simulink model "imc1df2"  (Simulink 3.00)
settings: Solver=ode45  SolverMode=SingleTasking  StartTime=0.0  StopTime=50  MaxStep=st_size  RelTol=1e-5  AbsTol=1e-6
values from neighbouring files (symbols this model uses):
  d_through_p = get(MAIN_MENU(19),'Value')    [cback.m]    (also in imcmenu.m = 0)
  Disturb = Setpoint    [mimo_MSF1DF_sim.m]    (also in mimo_MSF2DF_sim.m)
  Satlb = temp1    [cback.m]    (also in imcmenu.m = str2num(satlbs))
  Satub = temp1    [cback.m]    (also in imcmenu.m = str2num(satubs))
  Setpoint = zeros(1,n)    [mimo_MSF1DF_sim.m]    (also in mimo_MSF2DF_sim.m)
undefined symbols (not defined in the file or in its folder): denCs, denPd, mdeadx, numCs, numPd, pdeadx, XdenMs, XdenPs, XnumMs, XnumPs

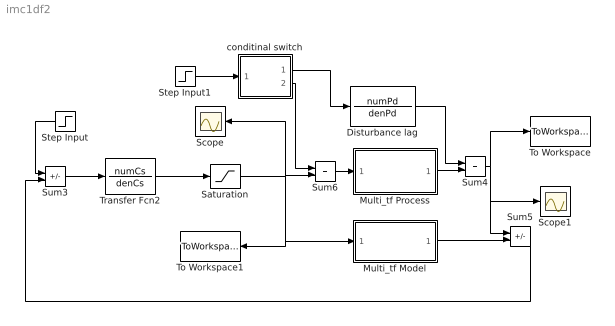
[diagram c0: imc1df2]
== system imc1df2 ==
  Disturbance lag : TransferFcn  Numerator=numPd  Denominator=denPd
  Multi_tf Model : Subsystem
  Multi_tf Process : Subsystem
  Saturation : Saturate  UpperLimit=Satub  LowerLimit=Satlb
  Scope : Scope
  Scope1 : Scope
  Step Input : Step  Orientation=left  Time=0  Before=0  After=Setpoint  SampleTime=0
  Step Input1 : Step  Time=0  Before=0  After=Disturb  SampleTime=0
  Sum3 : Sum  Inputs=+-  SaturateOnIntegerOverflow=on
  Sum4 : Sum  Inputs=++  SaturateOnIntegerOverflow=on
  Sum5 : Sum  Inputs=+-  SaturateOnIntegerOverflow=on
  Sum6 : Sum  Inputs=++  SaturateOnIntegerOverflow=on
  To Workspace : ToWorkspace  VariableName=simout  SampleTime=-1  SaveFormat=Matrix
  To Workspace1 : ToWorkspace  VariableName=effort  SampleTime=-1  SaveFormat=Matrix
  Transfer Fcn2 : TransferFcn  Numerator=numCs  Denominator=denCs
  conditinal switch : Subsystem  Description=pass input signal through out1 if condition is true.
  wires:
  Sum3/1 -> Transfer Fcn2/1
  Transfer Fcn2/1 -> Saturation/1
  Step Input/1 -> Sum3/1
  Sum5/1 -> Sum3/2
  Multi_tf Model/1(Out1) -> Sum5/2
  Disturbance lag/1 -> Sum4/1
  Step Input1/1 -> conditinal switch/1(In)
  conditinal switch/1(Out2) -> Disturbance lag/1
  Saturation/1 -> Sum6/2, Multi_tf Model/1(In1), Scope/1, To Workspace1/1
  conditinal switch/2(Out1) -> Sum6/1
  Sum6/1 -> Multi_tf Process/1(In1)
  Multi_tf Process/1(Out1) -> Sum4/2
  Sum4/1 -> Sum5/1, To Workspace/1, Scope1/1

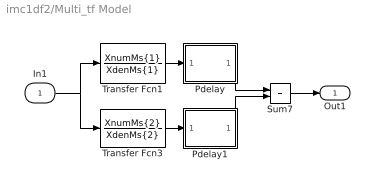
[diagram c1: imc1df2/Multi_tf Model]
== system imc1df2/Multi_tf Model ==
  In1 : Inport  Port=1  PortWidth=-1  SampleTime=-1  DataType=auto
  Pdelay : Subsystem
  Pdelay1 : Subsystem
  Sum7 : Sum  Inputs=++  SaturateOnIntegerOverflow=on
  Transfer Fcn1 : TransferFcn  Numerator=XnumMs{1}  Denominator=XdenMs{1}
  Transfer Fcn3 : TransferFcn  Numerator=XnumMs{2}  Denominator=XdenMs{2}
  Out1 : Outport  Port=1  InitialOutput=0
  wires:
  Transfer Fcn1/1 -> Pdelay/1(In1)
  Transfer Fcn3/1 -> Pdelay1/1(In1)
  In1/1 -> Transfer Fcn1/1, Transfer Fcn3/1
  Sum7/1 -> Out1/1
  Pdelay/1(Out1) -> Sum7/1
  Pdelay1/1(Out1) -> Sum7/2

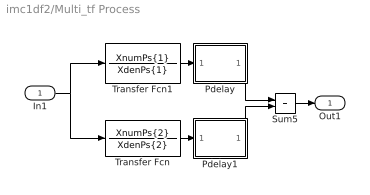
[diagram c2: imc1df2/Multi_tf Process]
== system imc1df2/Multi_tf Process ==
  In1 : Inport  Port=1  PortWidth=-1  SampleTime=-1  DataType=auto
  Pdelay : Subsystem
  Pdelay1 : Subsystem
  Sum5 : Sum  Inputs=++  SaturateOnIntegerOverflow=on
  Transfer Fcn : TransferFcn  Numerator=XnumPs{2}  Denominator=XdenPs{2}
  Transfer Fcn1 : TransferFcn  Numerator=XnumPs{1}  Denominator=XdenPs{1}
  Out1 : Outport  Port=1  InitialOutput=0
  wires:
  Transfer Fcn1/1 -> Pdelay/1(In1)
  Transfer Fcn/1 -> Pdelay1/1(In1)
  In1/1 -> Transfer Fcn1/1, Transfer Fcn/1
  Sum5/1 -> Out1/1
  Pdelay/1(Out1) -> Sum5/1
  Pdelay1/1(Out1) -> Sum5/2

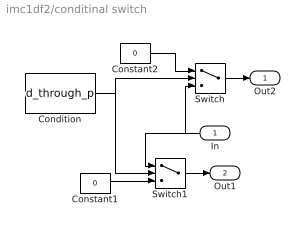
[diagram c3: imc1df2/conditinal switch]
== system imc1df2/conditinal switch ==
  In : Inport  Orientation=left  Port=1  PortWidth=-1  SampleTime=-1  DataType=auto
  Condition : Constant  Value=d_through_p
  Constant1 : Constant  Value=0
  Constant2 : Constant  Value=0
  Switch : Switch  Threshold=1
  Switch1 : Switch  Threshold=1
  Out2 : Outport  Port=1  InitialOutput=0
  Out1 : Outport  Port=2  InitialOutput=0
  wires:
  In/1 -> Switch/3, Switch1/1
  Condition/1 -> Switch1/2, Switch/2
  Constant1/1 -> Switch1/3
  Constant2/1 -> Switch/1
  Switch/1 -> Out2/1
  Switch1/1 -> Out1/1

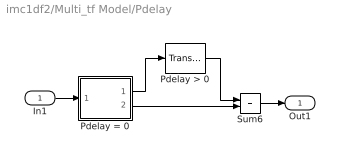
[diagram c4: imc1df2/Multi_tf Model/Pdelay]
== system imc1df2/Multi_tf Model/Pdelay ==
  In1 : Inport  Port=1  PortWidth=-1  SampleTime=-1  DataType=auto
  Pdelay > 0 : TransportDelay  DelayTime=mdeadx(1)  InitialInput=0  BufferSize=1024
  Pdelay = 0 : Subsystem  Description=pass input signal through out1 if condition is true.
  Sum6 : Sum  Inputs=++  SaturateOnIntegerOverflow=on
  Out1 : Outport  Port=1
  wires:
  Pdelay = 0/1(Out2) -> Pdelay > 0/1
  Pdelay > 0/1 -> Sum6/1
  Pdelay = 0/2(Out1) -> Sum6/2
  In1/1 -> Pdelay = 0/1(In)
  Sum6/1 -> Out1/1

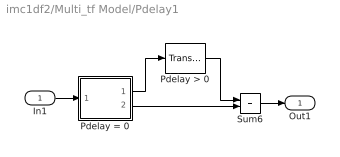
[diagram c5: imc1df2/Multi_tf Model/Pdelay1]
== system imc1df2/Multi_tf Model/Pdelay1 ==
  In1 : Inport  Port=1  PortWidth=-1  SampleTime=-1  DataType=auto
  Pdelay > 0 : TransportDelay  DelayTime=mdeadx(2)  InitialInput=0  BufferSize=1024
  Pdelay = 0 : Subsystem  Description=pass input signal through out1 if condition is true.
  Sum6 : Sum  Inputs=++  SaturateOnIntegerOverflow=on
  Out1 : Outport  Port=1
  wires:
  Pdelay = 0/1(Out2) -> Pdelay > 0/1
  Pdelay > 0/1 -> Sum6/1
  Pdelay = 0/2(Out1) -> Sum6/2
  In1/1 -> Pdelay = 0/1(In)
  Sum6/1 -> Out1/1

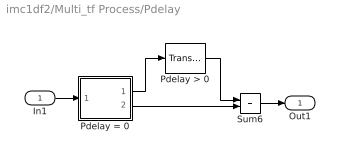
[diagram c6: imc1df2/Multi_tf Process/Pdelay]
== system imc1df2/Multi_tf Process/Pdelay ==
  In1 : Inport  Port=1  PortWidth=-1  SampleTime=-1  DataType=auto
  Pdelay > 0 : TransportDelay  DelayTime=pdeadx(1)  InitialInput=0  BufferSize=1024
  Pdelay = 0 : Subsystem  Description=pass input signal through out1 if condition is true.
  Sum6 : Sum  Inputs=++  SaturateOnIntegerOverflow=on
  Out1 : Outport  Port=1
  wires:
  Pdelay = 0/1(Out2) -> Pdelay > 0/1
  Pdelay > 0/1 -> Sum6/1
  Pdelay = 0/2(Out1) -> Sum6/2
  In1/1 -> Pdelay = 0/1(In)
  Sum6/1 -> Out1/1

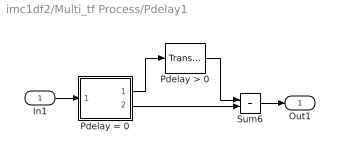
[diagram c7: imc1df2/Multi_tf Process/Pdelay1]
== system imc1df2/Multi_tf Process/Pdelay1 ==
  In1 : Inport  Port=1  PortWidth=-1  SampleTime=-1  DataType=auto
  Pdelay > 0 : TransportDelay  DelayTime=pdeadx(2)  InitialInput=0  BufferSize=1024
  Pdelay = 0 : Subsystem  Description=pass input signal through out1 if condition is true.
  Sum6 : Sum  Inputs=++  SaturateOnIntegerOverflow=on
  Out1 : Outport  Port=1
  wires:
  Pdelay = 0/1(Out2) -> Pdelay > 0/1
  Pdelay > 0/1 -> Sum6/1
  Pdelay = 0/2(Out1) -> Sum6/2
  In1/1 -> Pdelay = 0/1(In)
  Sum6/1 -> Out1/1

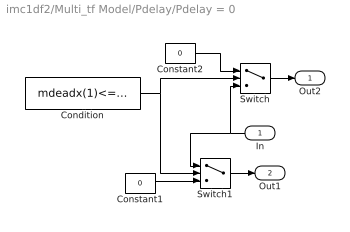
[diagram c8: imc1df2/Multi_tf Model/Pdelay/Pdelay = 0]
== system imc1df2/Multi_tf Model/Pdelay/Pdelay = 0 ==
  In : Inport  Orientation=left  Port=1  PortWidth=-1  SampleTime=-1  DataType=auto
  Condition : Constant  Value=mdeadx(1)<=3*eps
  Constant1 : Constant  Value=0
  Constant2 : Constant  Value=0
  Switch : Switch  Threshold=1
  Switch1 : Switch  Threshold=1
  Out2 : Outport  Port=1  InitialOutput=0
  Out1 : Outport  Port=2  InitialOutput=0
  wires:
  In/1 -> Switch/3, Switch1/1
  Condition/1 -> Switch1/2, Switch/2
  Constant1/1 -> Switch1/3
  Constant2/1 -> Switch/1
  Switch/1 -> Out2/1
  Switch1/1 -> Out1/1

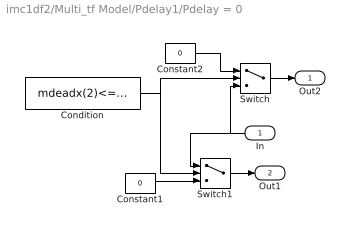
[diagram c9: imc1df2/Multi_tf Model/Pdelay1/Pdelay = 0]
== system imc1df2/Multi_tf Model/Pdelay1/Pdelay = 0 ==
  In : Inport  Orientation=left  Port=1  PortWidth=-1  SampleTime=-1  DataType=auto
  Condition : Constant  Value=mdeadx(2)<=3*eps
  Constant1 : Constant  Value=0
  Constant2 : Constant  Value=0
  Switch : Switch  Threshold=1
  Switch1 : Switch  Threshold=1
  Out2 : Outport  Port=1  InitialOutput=0
  Out1 : Outport  Port=2  InitialOutput=0
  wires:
  In/1 -> Switch/3, Switch1/1
  Condition/1 -> Switch1/2, Switch/2
  Constant1/1 -> Switch1/3
  Constant2/1 -> Switch/1
  Switch/1 -> Out2/1
  Switch1/1 -> Out1/1

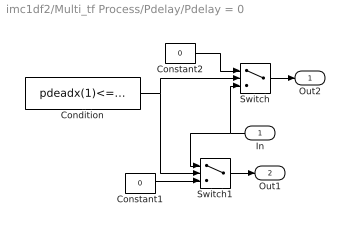
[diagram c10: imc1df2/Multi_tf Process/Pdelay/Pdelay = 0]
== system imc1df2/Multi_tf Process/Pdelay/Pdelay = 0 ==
  In : Inport  Orientation=left  Port=1  PortWidth=-1  SampleTime=-1  DataType=auto
  Condition : Constant  Value=pdeadx(1)<=3*eps
  Constant1 : Constant  Value=0
  Constant2 : Constant  Value=0
  Switch : Switch  Threshold=1
  Switch1 : Switch  Threshold=1
  Out2 : Outport  Port=1  InitialOutput=0
  Out1 : Outport  Port=2  InitialOutput=0
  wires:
  In/1 -> Switch/3, Switch1/1
  Condition/1 -> Switch1/2, Switch/2
  Constant1/1 -> Switch1/3
  Constant2/1 -> Switch/1
  Switch/1 -> Out2/1
  Switch1/1 -> Out1/1

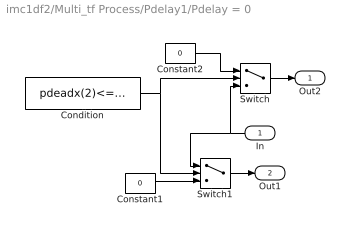
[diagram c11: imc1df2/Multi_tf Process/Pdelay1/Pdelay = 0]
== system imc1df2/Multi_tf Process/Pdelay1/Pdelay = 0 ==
  In : Inport  Orientation=left  Port=1  PortWidth=-1  SampleTime=-1  DataType=auto
  Condition : Constant  Value=pdeadx(2)<=3*eps
  Constant1 : Constant  Value=0
  Constant2 : Constant  Value=0
  Switch : Switch  Threshold=1
  Switch1 : Switch  Threshold=1
  Out2 : Outport  Port=1  InitialOutput=0
  Out1 : Outport  Port=2  InitialOutput=0
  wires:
  In/1 -> Switch/3, Switch1/1
  Condition/1 -> Switch1/2, Switch/2
  Constant1/1 -> Switch1/3
  Constant2/1 -> Switch/1
  Switch/1 -> Out2/1
  Switch1/1 -> Out1/1
